(* Logix 5000 AddOnInstructionDefinition export YAI_Assy_166_120_EIP_Hz; software revision 21.03 *)

ADD_ON_INSTRUCTION YAI_Assy_166_120_EIP_Hz   (* revision 1.1, vendor Yaskawa America, Inc. *)
// YAI Assembly 166 and 120
// Revision note:
// Corrected Custom_Out_x function.
// Help:
// This add-on instruction is for use with input assemblie 166 and output assemblies 120.
// Node_Input_Assy is defined as the node's input assembly integer array.
// Node_Output_Assy is defined as the node's output assembly integer array.
// Torque limit/reference, torque compensation and torque output variables are only available with A1000.
VAR_IN_OUT
   Node_Input_Assy : AB:ETHERNET_MODULE_INT_44Bytes:I:0; {required}   // Input assembly words
   Node_Output_Assy : AB:ETHERNET_MODULE_INT_24Bytes:I:0; {required}   // Output assembly words
END_VAR
VAR_INPUT
   RunFwd : BOOL; {visible}   // Forward run command
   RunRev : BOOL; {visible}   // Reverse run command
   MFI_3 : BOOL; {visible}   // Multi-function input 3
   MFI_4 : BOOL; {visible}   // Multi-function input 4
   MFI_5 : BOOL; {visible}   // Multi-function input 5
   MFI_6 : BOOL; {visible}   // Multi-function input 6
   MFI_7 : BOOL; {visible}   // Multi-function input 7
   MFI_8 : BOOL; {visible}   // Multi-function input 8
   External_Fault : BOOL;   // External fault command (EF0)
   FaultReset : BOOL; {visible}   // Fault reset command
   MFO_1 : BOOL; {visible}   // Multi-function output (M1-M2 for A/P1000, MA/MB/MC for V1000)
   MFO_2 : BOOL; {visible}   // Multi-function output (M3-M4 for A/P1000, P1 for V1000)
   MFO_3 : BOOL; {visible}   // Multi-function output (M5-M6 for A/P1000, P2 for V1000)
   Freq_Ref : REAL; {visible}   // Frequency reference command in Hz (xx.xx resolution)
   Net_Ref : BOOL;   // Network reference control bit
   Net_Control : BOOL;   // Network start/stop control bit
   Custom_Out_1 : INT; {visible}   // Custom output 1 - F7-23
   Custom_Out_2 : INT; {visible}   // Custom output 2 - F7-24
   Custom_Out_3 : INT; {visible}   // Custom output 3 - F7-25
   Custom_Out_4 : INT;   // Custom output 4 - F7-26
   Custom_Out_5 : INT;   // Custom output 5 - F7-27
   Custom_Out_6 : INT;   // Custom output 6 - F7-28
   Custom_Out_7 : INT;   // Custom output 7 - F7-29
   Custom_Out_8 : INT;   // Custom output 8 - F7-30
   Custom_Out_9 : INT;   // Custom output 9 - F7-31
   Custom_Out_10 : INT;   // Custom output 10 - F7-32
END_VAR
VAR_OUTPUT
   Running : BOOL; {access Read Only, visible}   // Drive running forward status bit
   ZSP : BOOL; {access Read Only, visible}   // Drive zero speed status bit
   RunningRev : BOOL; {access Read Only, visible}   // Drive running reverse status bit
   Reset : BOOL; {access Read Only, visible}   // Drive reset command status bit
   At_Speed : BOOL; {access Read Only, visible}   // Drive at commanded speed status bit
   Ready : BOOL; {access Read Only, visible}   // Drive ready status bit
   Alarm : BOOL; {access Read Only, visible}   // Drive alarm status bit
   Faulted : BOOL; {access Read Only, visible}   // Drive faulted status bit
   OPE : BOOL; {access Read Only}   // OPE alarm/fault present
   UV : BOOL; {access Read Only}   // Drive in UV (undervoltage) state status bit
   NetCtrlStatus : BOOL; {access Read Only, visible}   // Drive network run source status bit (1 = source coming from network)
   MFO_1_Status : BOOL; {access Read Only, visible}   // Drive multi-function output 1 (M1-M2 for A/P1000, MA/MB/MC for V1000) status
   MFO_2_Status : BOOL; {access Read Only, visible}   // Drive multi-function output 1 (M3-M4 for A/P1000, P1 for V1000) status
   MFO_3_Status : BOOL; {access Read Only, visible}   // Drive multi-function output 1 (M5-M6 for A/P1000, P2 for V1000) status
   ZSV : BOOL; {access Read Only, visible}   // Drive zero servo completed status bit
   Motor_Speed : REAL; {access Read Only, visible}   // Motor speed in Hz (xx.xx resolution)
   Torque_Actual : REAL; {access Read Only, visible}   // Drive torque output in % (xxx.x resolution)
   PG_Count : INT; {access Read Only}   // Encoder feedback count
   Freq_Cmd : REAL; {access Read Only, visible}   // Commanded frequency in Hz (xx.xx resolution)
   Output_Freq : REAL; {access Read Only, visible}   // Drive output frequency in Hz (xx.xx resolution)
   Output_Current : REAL; {access Read Only, visible}   // Drive output current in A (xxx.x resolution)
   Analog_Input_1_Level : REAL; {access Read Only}   // Analog input 1 level in % (xxx.x resolution)
   DC_Bus_Volt : INT; {access Read Only, visible}   // DC bus voltage in Vdc (xxx resolution)
   Error_Code : INT; {access Read Only}   // Custom input/output error code. Refer to custom error bit to determine which parameter error is pertaining to.
   Custom_In_1 : INT; {access Read Only, visible}   // Custom input 1 - F7-33
   Custom_In_2 : INT; {access Read Only, visible}   // Custom input 2 - F7-34
   Custom_In_3 : INT; {access Read Only, visible}   // Custom input 3 - F7-35
   Custom_In_4 : INT; {access Read Only}   // Custom input 4 - F7-36
   Custom_In_5 : INT; {access Read Only}   // Custom input 5 - F7-37
   Custom_In_6 : INT; {access Read Only}   // Custom input 6 - F7-38
   Custom_In_7 : INT; {access Read Only}   // Custom input 7 - F7-39
   Custom_In_8 : INT; {access Read Only}   // Custom input 8 -F7-40
   Custom_In_9 : INT; {access Read Only}   // Custom input 9 - F7-41
   Custom_In_10 : INT; {access Read Only}   // Custom input 10 - F7-42
   Custom_Out_1_Error : BOOL; {access Read Only}   // Custom output 1 error bit
   Custom_Out_2_Error : BOOL; {access Read Only}   // Custom output 2 error bit
   Custom_Out_3_Error : BOOL; {access Read Only}   // Custom output 3 error bit
   Custom_Out_4_Error : BOOL; {access Read Only}   // Custom output 4 error bit
   Custom_Out_5_Error : BOOL; {access Read Only}   // Custom output 5 error bit
   Custom_Out_6_Error : BOOL; {access Read Only}   // Custom output 6 error bit
   Custom_Out_7_Error : BOOL; {access Read Only}   // Custom output 7 error bit
   Custom_Out_8_Error : BOOL; {access Read Only}   // Custom output 8 error bit
   Custom_Out_9_Error : BOOL; {access Read Only}   // Custom output 9 error bit
   Custom_Out_10_Error : BOOL; {access Read Only}   // Custom output 10 error bit
   Custom_In_1_Error : BOOL; {access Read Only}   // Custom input 1 error bit
   Custom_In_2_Error : BOOL; {access Read Only}   // Custom input 2 error bit
   Custom_In_3_Error : BOOL; {access Read Only}   // Custom input 3 error bit
   Custom_In_4_Error : BOOL; {access Read Only}   // Custom input 4 error bit
   Custom_In_5_Error : BOOL; {access Read Only}   // Custom input 5 error bit
   Custom_In_6_Error : BOOL; {access Read Only}   // Custom input 6 error bit
   Custom_In_7_Error : BOOL; {access Read Only}   // Custom input 7 error bit
   Custom_In_8_Error : BOOL; {access Read Only}   // Custom input 8 error bit
   Custom_In_9_Error : BOOL; {access Read Only}   // Custom input 9 error bit
   Custom_In_10_Error : BOOL; {access Read Only}   // Custom input 10 error bit
END_VAR
VAR
   FRef_Convert : DINT;
   FOut_Convert : REAL;
   FOut_Temp : REAL;
   TRef_Convert : INT;
   TComp_Convert : INT;
   TOut_Convert : REAL;
   TOut_Temp : REAL;
   IOut_Temp : REAL;
   IOut_Convert : REAL;
   AO1_Convert : INT;
   AO2_Convert : INT;
   Motor_Speed_Temp : REAL;
   Motor_Speed_Convert : REAL;
   Freq_Cmd_Temp : REAL;
   Freq_Cmd_Convert : REAL;
   AI1_Temp : REAL;
   AI1_Convert : REAL;
END_VAR

ROUTINE Logic   (* ladder *)
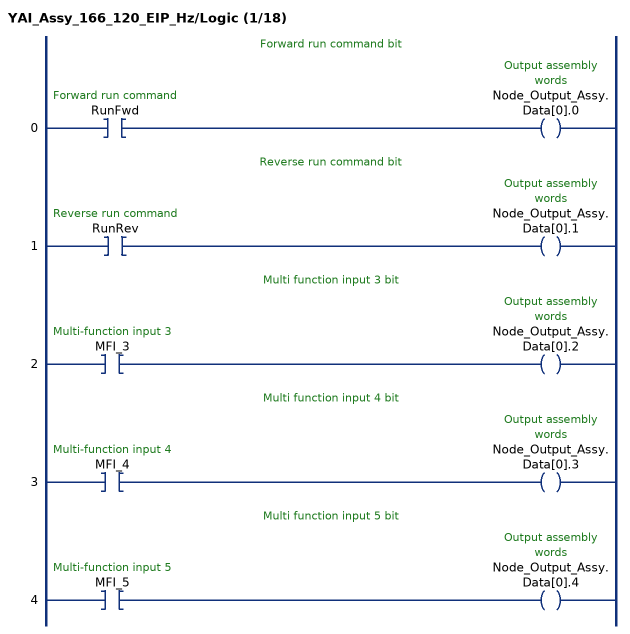
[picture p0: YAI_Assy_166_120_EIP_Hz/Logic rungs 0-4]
   // Forward run command bit
   0: XIC(RunFwd)OTE(Node_Output_Assy.Data[0].0);
   // Reverse run command bit
   1: XIC(RunRev)OTE(Node_Output_Assy.Data[0].1);
   // Multi function input 3 bit
   2: XIC(MFI_3)OTE(Node_Output_Assy.Data[0].2);
   // Multi function input 4 bit
   3: XIC(MFI_4)OTE(Node_Output_Assy.Data[0].3);
   // Multi function input 5 bit
   4: XIC(MFI_5)OTE(Node_Output_Assy.Data[0].4);
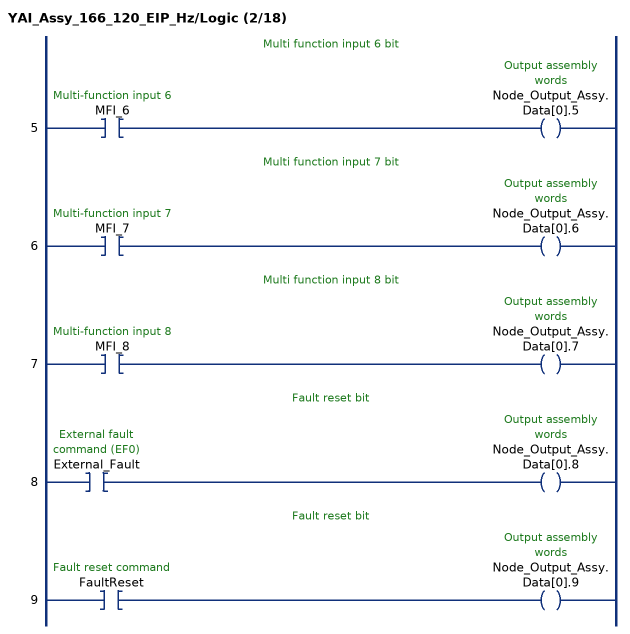
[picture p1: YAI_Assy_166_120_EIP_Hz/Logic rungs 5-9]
   // Multi function input 6 bit
   5: XIC(MFI_6)OTE(Node_Output_Assy.Data[0].5);
   // Multi function input 7 bit
   6: XIC(MFI_7)OTE(Node_Output_Assy.Data[0].6);
   // Multi function input 8 bit
   7: XIC(MFI_8)OTE(Node_Output_Assy.Data[0].7);
   // Fault reset bit
   8: XIC(External_Fault)OTE(Node_Output_Assy.Data[0].8);
   // Fault reset bit
   9: XIC(FaultReset)OTE(Node_Output_Assy.Data[0].9);
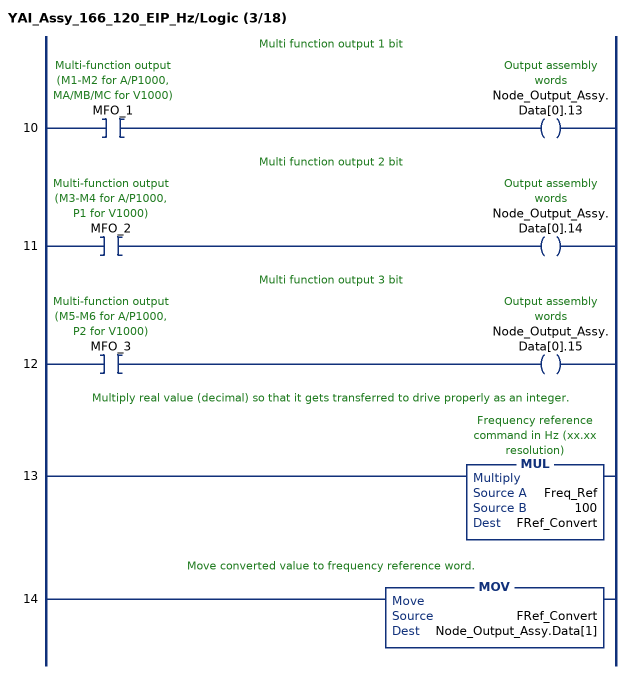
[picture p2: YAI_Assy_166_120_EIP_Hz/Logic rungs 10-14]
   // Multi function output 1 bit
   10: XIC(MFO_1)OTE(Node_Output_Assy.Data[0].13);
   // Multi function output 2 bit
   11: XIC(MFO_2)OTE(Node_Output_Assy.Data[0].14);
   // Multi function output 3 bit
   12: XIC(MFO_3)OTE(Node_Output_Assy.Data[0].15);
   // Multiply real value (decimal) so that it gets transferred to drive properly as an integer.
   13: MUL(Freq_Ref,100,FRef_Convert);
   // Move converted value to frequency reference word.
   14: MOV(FRef_Convert,Node_Output_Assy.Data[1]);
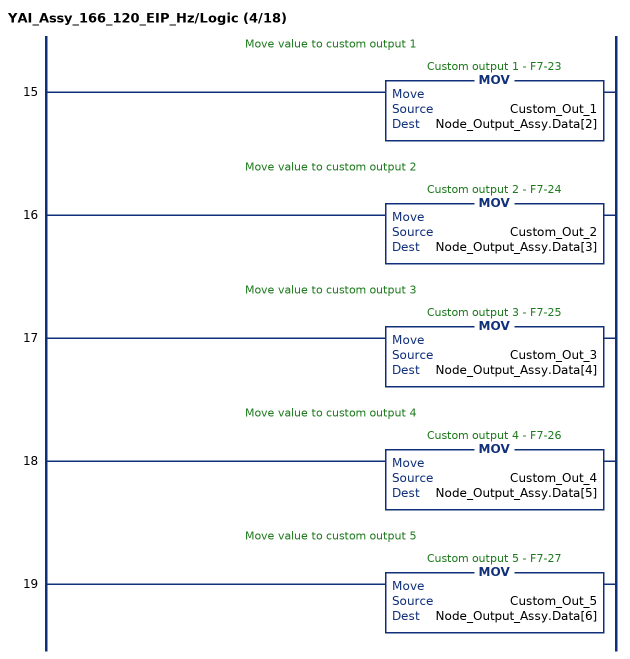
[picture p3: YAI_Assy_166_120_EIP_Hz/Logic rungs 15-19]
   // Move value to custom output 1
   15: MOV(Custom_Out_1,Node_Output_Assy.Data[2]);
   // Move value to custom output 2
   16: MOV(Custom_Out_2,Node_Output_Assy.Data[3]);
   // Move value to custom output 3
   17: MOV(Custom_Out_3,Node_Output_Assy.Data[4]);
   // Move value to custom output 4
   18: MOV(Custom_Out_4,Node_Output_Assy.Data[5]);
   // Move value to custom output 5
   19: MOV(Custom_Out_5,Node_Output_Assy.Data[6]);
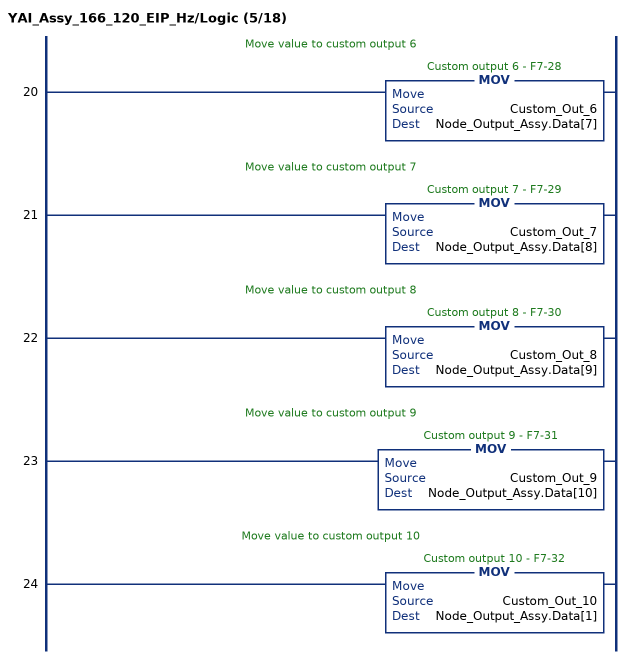
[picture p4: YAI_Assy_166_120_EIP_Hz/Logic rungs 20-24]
   // Move value to custom output 6
   20: MOV(Custom_Out_6,Node_Output_Assy.Data[7]);
   // Move value to custom output 7
   21: MOV(Custom_Out_7,Node_Output_Assy.Data[8]);
   // Move value to custom output 8
   22: MOV(Custom_Out_8,Node_Output_Assy.Data[9]);
   // Move value to custom output 9
   23: MOV(Custom_Out_9,Node_Output_Assy.Data[10]);
   // Move value to custom output 10
   24: MOV(Custom_Out_10,Node_Output_Assy.Data[1]);
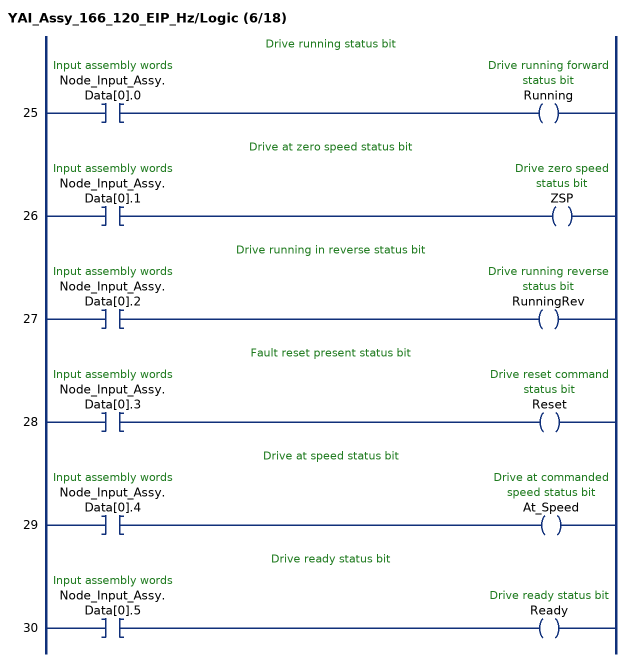
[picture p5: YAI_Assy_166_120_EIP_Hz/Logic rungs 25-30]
   // Drive running status bit
   25: XIC(Node_Input_Assy.Data[0].0)OTE(Running);
   // Drive at zero speed status bit
   26: XIC(Node_Input_Assy.Data[0].1)OTE(ZSP);
   // Drive running in reverse status bit
   27: XIC(Node_Input_Assy.Data[0].2)OTE(RunningRev);
   // Fault reset present status bit
   28: XIC(Node_Input_Assy.Data[0].3)OTE(Reset);
   // Drive at speed status bit
   29: XIC(Node_Input_Assy.Data[0].4)OTE(At_Speed);
   // Drive ready status bit
   30: XIC(Node_Input_Assy.Data[0].5)OTE(Ready);
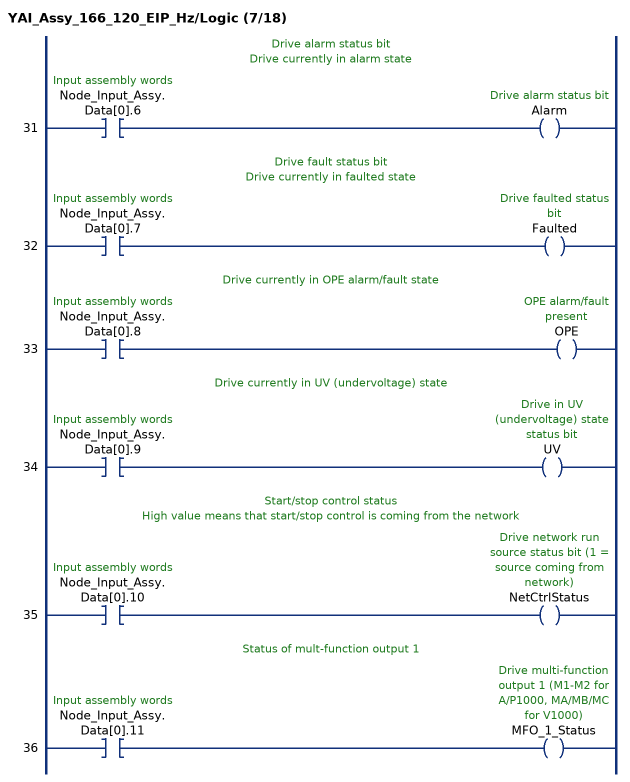
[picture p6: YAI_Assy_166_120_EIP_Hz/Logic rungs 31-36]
   // Drive alarm status bit
   // Drive currently in alarm state
   31: XIC(Node_Input_Assy.Data[0].6)OTE(Alarm);
   // Drive fault status bit
   // Drive currently in faulted state
   32: XIC(Node_Input_Assy.Data[0].7)OTE(Faulted);
   // Drive currently in OPE alarm/fault state
   33: XIC(Node_Input_Assy.Data[0].8)OTE(OPE);
   // Drive currently in UV (undervoltage) state
   34: XIC(Node_Input_Assy.Data[0].9)OTE(UV);
   // Start/stop control status
   // High value means that start/stop control is coming from the network
   35: XIC(Node_Input_Assy.Data[0].10)OTE(NetCtrlStatus);
   // Status of mult-function output 1
   36: XIC(Node_Input_Assy.Data[0].11)OTE(MFO_1_Status);
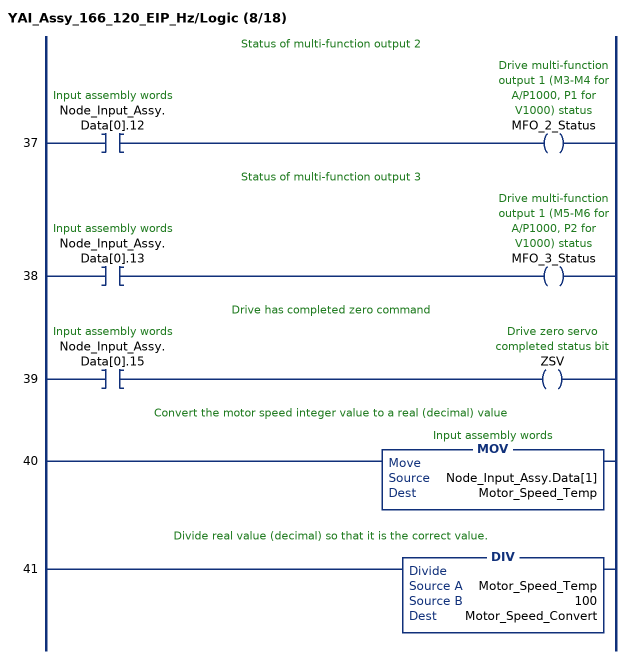
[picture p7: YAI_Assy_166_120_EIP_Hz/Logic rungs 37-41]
   // Status of multi-function output 2
   37: XIC(Node_Input_Assy.Data[0].12)OTE(MFO_2_Status);
   // Status of multi-function output 3
   38: XIC(Node_Input_Assy.Data[0].13)OTE(MFO_3_Status);
   // Drive has completed zero command
   39: XIC(Node_Input_Assy.Data[0].15)OTE(ZSV);
   // Convert the motor speed integer value to a real (decimal) value
   40: MOV(Node_Input_Assy.Data[1],Motor_Speed_Temp);
   // Divide real value (decimal) so that it is the correct value.
   41: DIV(Motor_Speed_Temp,100,Motor_Speed_Convert);
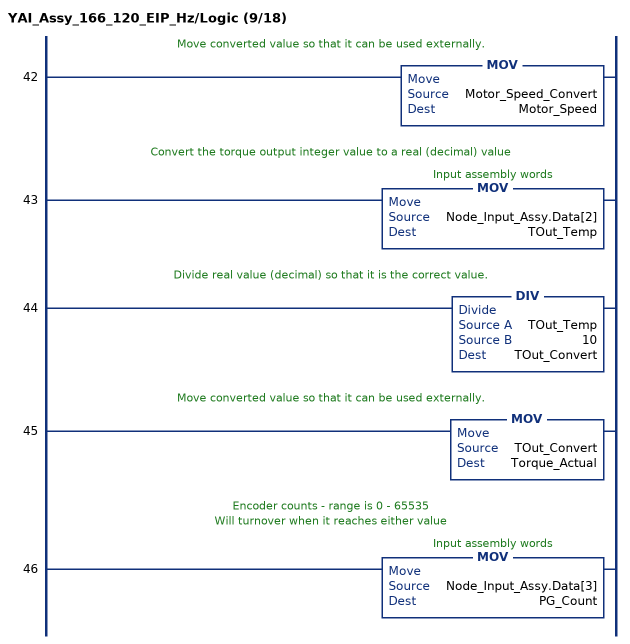
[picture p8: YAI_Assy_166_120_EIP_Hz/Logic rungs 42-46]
   // Move converted value so that it can be used externally.
   42: MOV(Motor_Speed_Convert,Motor_Speed);
   // Convert the torque output integer value to a real (decimal) value
   43: MOV(Node_Input_Assy.Data[2],TOut_Temp);
   // Divide real value (decimal) so that it is the correct value.
   44: DIV(TOut_Temp,10,TOut_Convert);
   // Move converted value so that it can be used externally.
   45: MOV(TOut_Convert,Torque_Actual);
   // Encoder counts - range is 0 - 65535
   // Will turnover when it reaches either value
   46: MOV(Node_Input_Assy.Data[3],PG_Count);
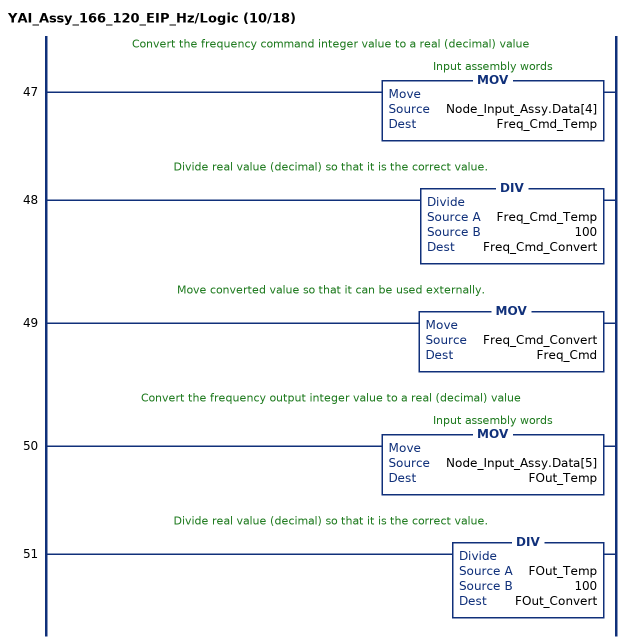
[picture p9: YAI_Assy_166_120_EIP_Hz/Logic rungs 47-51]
   // Convert the frequency command integer value to a real (decimal) value
   47: MOV(Node_Input_Assy.Data[4],Freq_Cmd_Temp);
   // Divide real value (decimal) so that it is the correct value.
   48: DIV(Freq_Cmd_Temp,100,Freq_Cmd_Convert);
   // Move converted value so that it can be used externally.
   49: MOV(Freq_Cmd_Convert,Freq_Cmd);
   // Convert the frequency output integer value to a real (decimal) value
   50: MOV(Node_Input_Assy.Data[5],FOut_Temp);
   // Divide real value (decimal) so that it is the correct value.
   51: DIV(FOut_Temp,100,FOut_Convert);
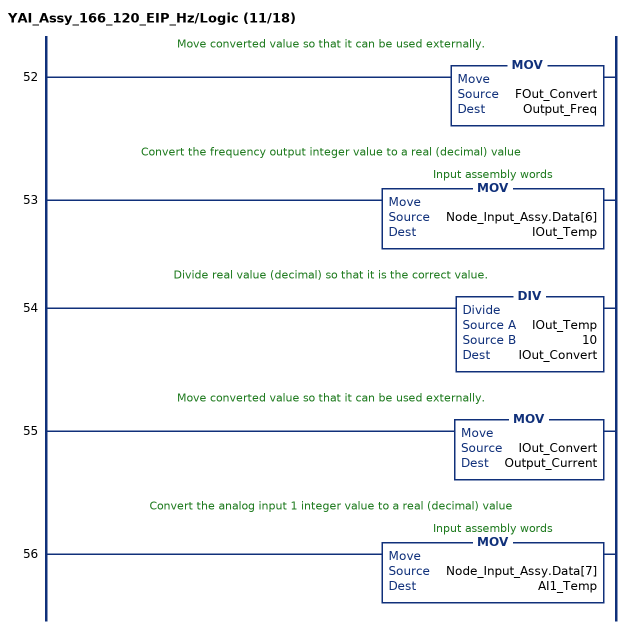
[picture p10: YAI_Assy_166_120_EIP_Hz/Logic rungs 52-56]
   // Move converted value so that it can be used externally.
   52: MOV(FOut_Convert,Output_Freq);
   // Convert the frequency output integer value to a real (decimal) value
   53: MOV(Node_Input_Assy.Data[6],IOut_Temp);
   // Divide real value (decimal) so that it is the correct value.
   54: DIV(IOut_Temp,10,IOut_Convert);
   // Move converted value so that it can be used externally.
   55: MOV(IOut_Convert,Output_Current);
   // Convert the analog input 1 integer value to a real (decimal) value
   56: MOV(Node_Input_Assy.Data[7],AI1_Temp);
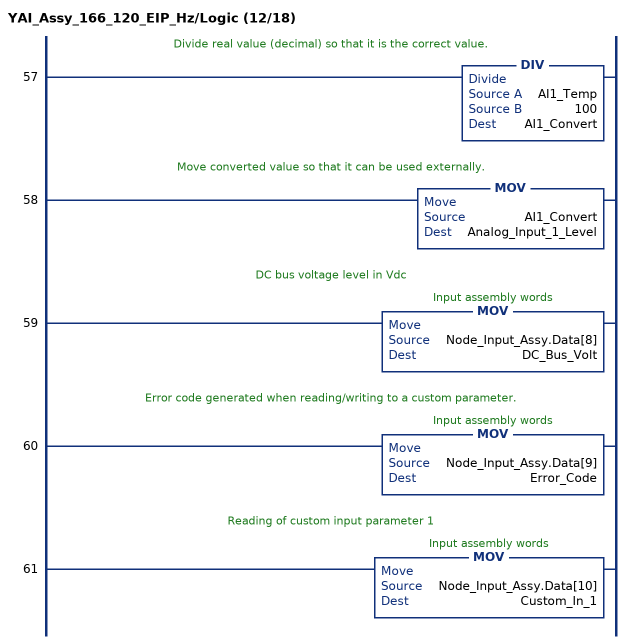
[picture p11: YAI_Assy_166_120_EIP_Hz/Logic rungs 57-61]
   // Divide real value (decimal) so that it is the correct value.
   57: DIV(AI1_Temp,100,AI1_Convert);
   // Move converted value so that it can be used externally.
   58: MOV(AI1_Convert,Analog_Input_1_Level);
   // DC bus voltage level in Vdc
   59: MOV(Node_Input_Assy.Data[8],DC_Bus_Volt);
   // Error code generated when reading/writing to a custom parameter.
   60: MOV(Node_Input_Assy.Data[9],Error_Code);
   // Reading of custom input parameter 1
   61: MOV(Node_Input_Assy.Data[10],Custom_In_1);
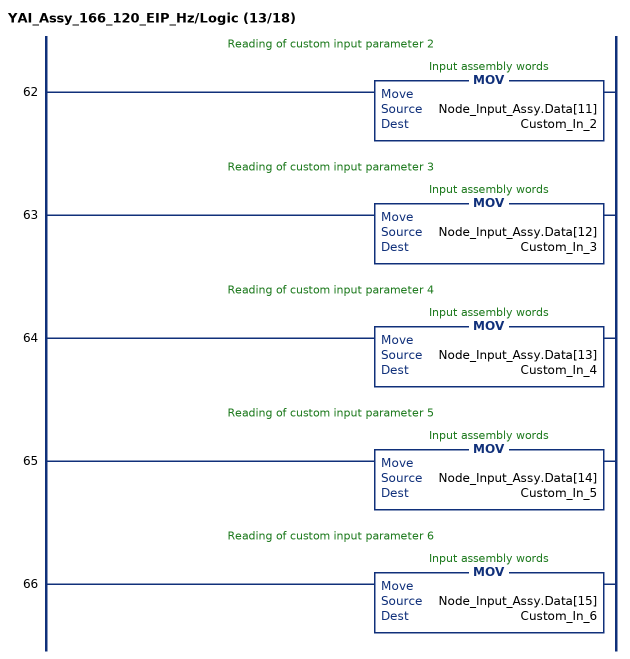
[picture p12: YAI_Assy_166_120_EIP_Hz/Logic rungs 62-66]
   // Reading of custom input parameter 2
   62: MOV(Node_Input_Assy.Data[11],Custom_In_2);
   // Reading of custom input parameter 3
   63: MOV(Node_Input_Assy.Data[12],Custom_In_3);
   // Reading of custom input parameter 4
   64: MOV(Node_Input_Assy.Data[13],Custom_In_4);
   // Reading of custom input parameter 5
   65: MOV(Node_Input_Assy.Data[14],Custom_In_5);
   // Reading of custom input parameter 6
   66: MOV(Node_Input_Assy.Data[15],Custom_In_6);
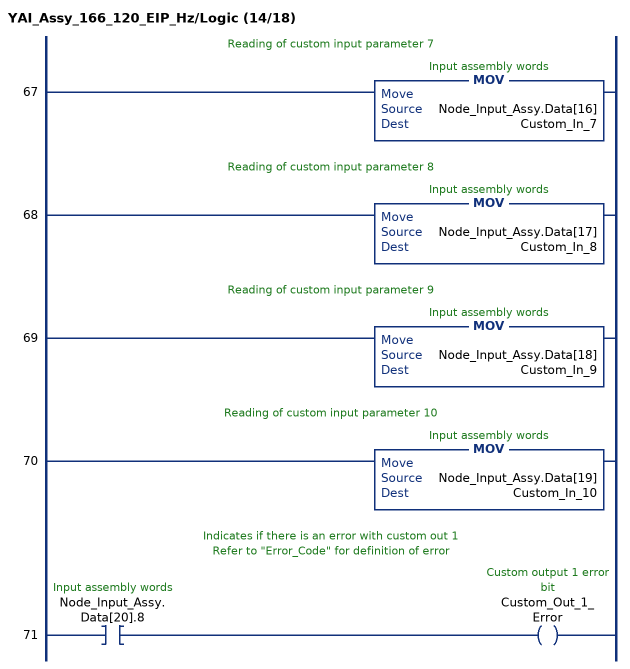
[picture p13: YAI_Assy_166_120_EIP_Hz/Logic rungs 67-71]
   // Reading of custom input parameter 7
   67: MOV(Node_Input_Assy.Data[16],Custom_In_7);
   // Reading of custom input parameter 8
   68: MOV(Node_Input_Assy.Data[17],Custom_In_8);
   // Reading of custom input parameter 9
   69: MOV(Node_Input_Assy.Data[18],Custom_In_9);
   // Reading of custom input parameter 10
   70: MOV(Node_Input_Assy.Data[19],Custom_In_10);
   // Indicates if there is an error with custom out 1
   // Refer to "Error_Code" for definition of error
   71: XIC(Node_Input_Assy.Data[20].8)OTE(Custom_Out_1_Error);
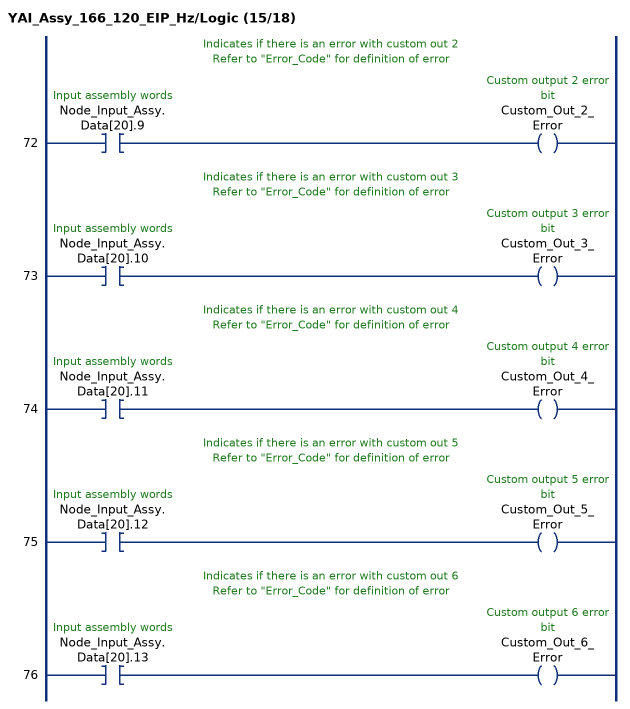
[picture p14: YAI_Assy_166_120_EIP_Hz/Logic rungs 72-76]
   // Indicates if there is an error with custom out 2
   // Refer to "Error_Code" for definition of error
   72: XIC(Node_Input_Assy.Data[20].9)OTE(Custom_Out_2_Error);
   // Indicates if there is an error with custom out 3
   // Refer to "Error_Code" for definition of error
   73: XIC(Node_Input_Assy.Data[20].10)OTE(Custom_Out_3_Error);
   // Indicates if there is an error with custom out 4
   // Refer to "Error_Code" for definition of error
   74: XIC(Node_Input_Assy.Data[20].11)OTE(Custom_Out_4_Error);
   // Indicates if there is an error with custom out 5
   // Refer to "Error_Code" for definition of error
   75: XIC(Node_Input_Assy.Data[20].12)OTE(Custom_Out_5_Error);
   // Indicates if there is an error with custom out 6
   // Refer to "Error_Code" for definition of error
   76: XIC(Node_Input_Assy.Data[20].13)OTE(Custom_Out_6_Error);
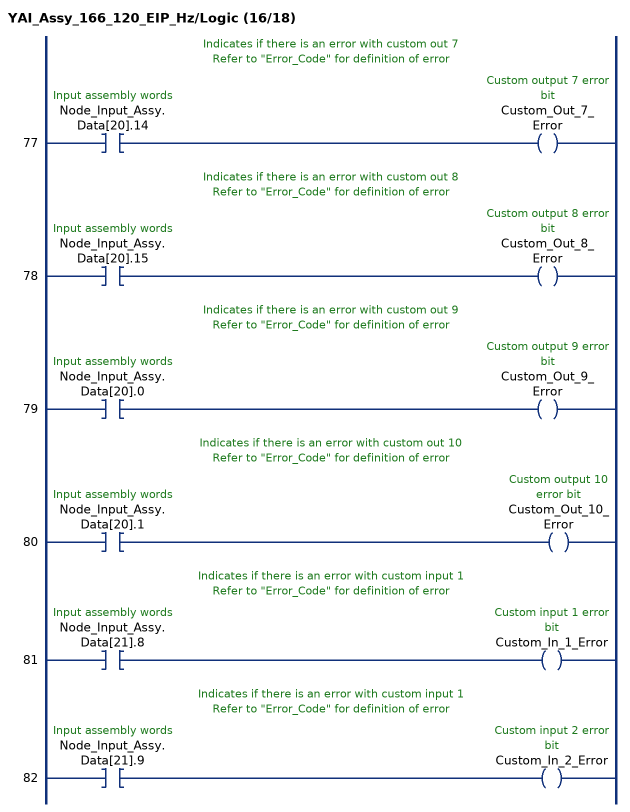
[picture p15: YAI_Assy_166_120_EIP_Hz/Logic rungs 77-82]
   // Indicates if there is an error with custom out 7
   // Refer to "Error_Code" for definition of error
   77: XIC(Node_Input_Assy.Data[20].14)OTE(Custom_Out_7_Error);
   // Indicates if there is an error with custom out 8
   // Refer to "Error_Code" for definition of error
   78: XIC(Node_Input_Assy.Data[20].15)OTE(Custom_Out_8_Error);
   // Indicates if there is an error with custom out 9
   // Refer to "Error_Code" for definition of error
   79: XIC(Node_Input_Assy.Data[20].0)OTE(Custom_Out_9_Error);
   // Indicates if there is an error with custom out 10
   // Refer to "Error_Code" for definition of error
   80: XIC(Node_Input_Assy.Data[20].1)OTE(Custom_Out_10_Error);
   // Indicates if there is an error with custom input 1
   // Refer to "Error_Code" for definition of error
   81: XIC(Node_Input_Assy.Data[21].8)OTE(Custom_In_1_Error);
   // Indicates if there is an error with custom input 1
   // Refer to "Error_Code" for definition of error
   82: XIC(Node_Input_Assy.Data[21].9)OTE(Custom_In_2_Error);
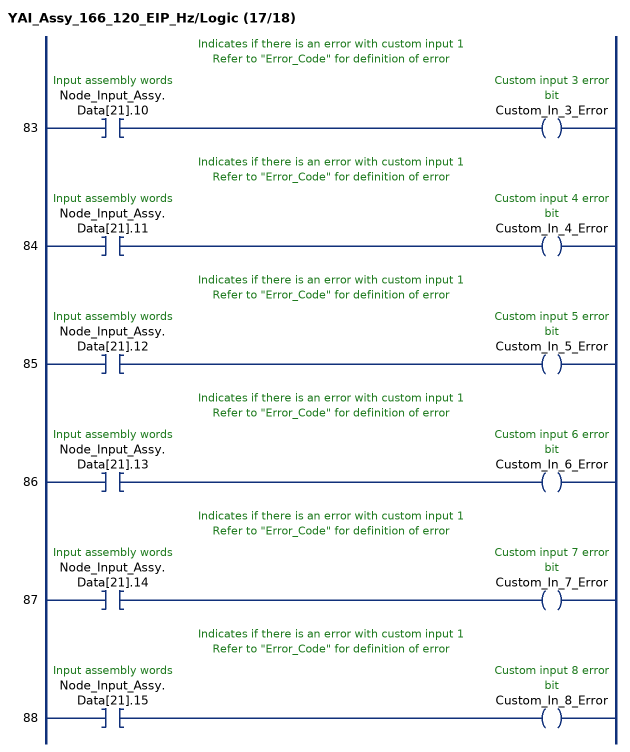
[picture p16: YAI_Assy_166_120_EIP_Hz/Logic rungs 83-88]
   // Indicates if there is an error with custom input 1
   // Refer to "Error_Code" for definition of error
   83: XIC(Node_Input_Assy.Data[21].10)OTE(Custom_In_3_Error);
   // Indicates if there is an error with custom input 1
   // Refer to "Error_Code" for definition of error
   84: XIC(Node_Input_Assy.Data[21].11)OTE(Custom_In_4_Error);
   // Indicates if there is an error with custom input 1
   // Refer to "Error_Code" for definition of error
   85: XIC(Node_Input_Assy.Data[21].12)OTE(Custom_In_5_Error);
   // Indicates if there is an error with custom input 1
   // Refer to "Error_Code" for definition of error
   86: XIC(Node_Input_Assy.Data[21].13)OTE(Custom_In_6_Error);
   // Indicates if there is an error with custom input 1
   // Refer to "Error_Code" for definition of error
   87: XIC(Node_Input_Assy.Data[21].14)OTE(Custom_In_7_Error);
   // Indicates if there is an error with custom input 1
   // Refer to "Error_Code" for definition of error
   88: XIC(Node_Input_Assy.Data[21].15)OTE(Custom_In_8_Error);
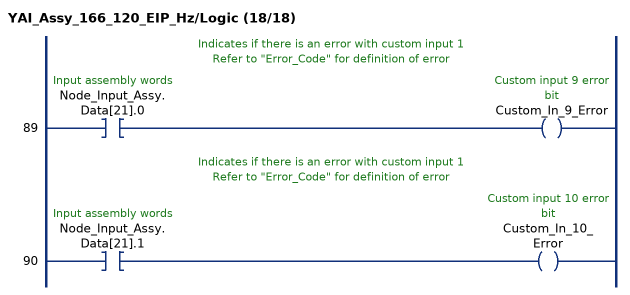
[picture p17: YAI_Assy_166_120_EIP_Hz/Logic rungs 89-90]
   // Indicates if there is an error with custom input 1
   // Refer to "Error_Code" for definition of error
   89: XIC(Node_Input_Assy.Data[21].0)OTE(Custom_In_9_Error);
   // Indicates if there is an error with custom input 1
   // Refer to "Error_Code" for definition of error
   90: XIC(Node_Input_Assy.Data[21].1)OTE(Custom_In_10_Error);
END_ROUTINE
END_ADD_ON_INSTRUCTION
